FUNCTION FC 23 : VOID
TITLE =USCITE E COMANDI BANCO DI SCARICO
VERSION : 0.1

BEGIN
NETWORK
TITLE =AVANTI BATTUTA NASTRO SCARICO
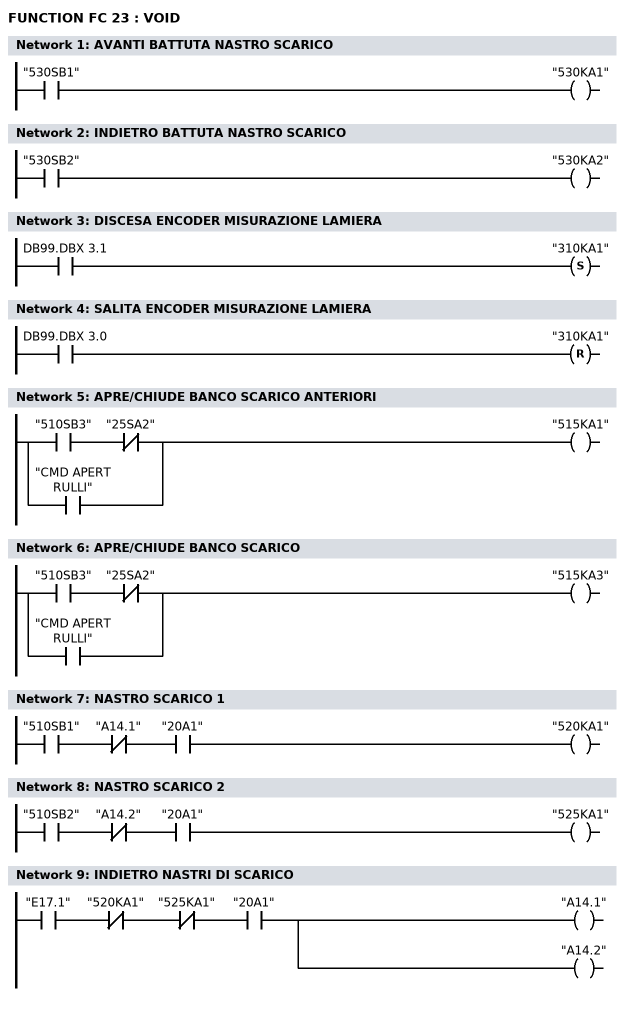
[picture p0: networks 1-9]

      U     "530SB1";
      =     "530KA1";
NETWORK
TITLE =INDIETRO BATTUTA NASTRO SCARICO

      U     "530SB2";
      =     "530KA2";
NETWORK
TITLE =DISCESA ENCODER MISURAZIONE LAMIERA

      U     DB99.DBX    3.1;
      S     "310KA1";
NETWORK
TITLE =SALITA ENCODER MISURAZIONE LAMIERA

      U     DB99.DBX    3.0;
      R     "310KA1";
NETWORK
TITLE =APRE/CHIUDE BANCO SCARICO ANTERIORI

      U     "510SB3";
      UN    "25SA2";
      O     "CMD APERT RULLI";
      =     "515KA1";
NETWORK
TITLE =APRE/CHIUDE BANCO SCARICO

      U     "510SB3";
      UN    "25SA2";
      O     "CMD APERT RULLI";
      =     "515KA3";
NETWORK
TITLE =NASTRO SCARICO 1

      U     "510SB1";
      UN    "A14.1";
      U     "20A1";
      =     "520KA1";
NETWORK
TITLE =NASTRO SCARICO 2

      U     "510SB2";
      UN    "A14.2";
      U     "20A1";
      =     "525KA1";
NETWORK
TITLE =INDIETRO NASTRI DI SCARICO

      U     "E17.1";
      UN    "520KA1";
      UN    "525KA1";
      U     "20A1";
      =     "A14.1";
      =     "A14.2";
END_FUNCTION

